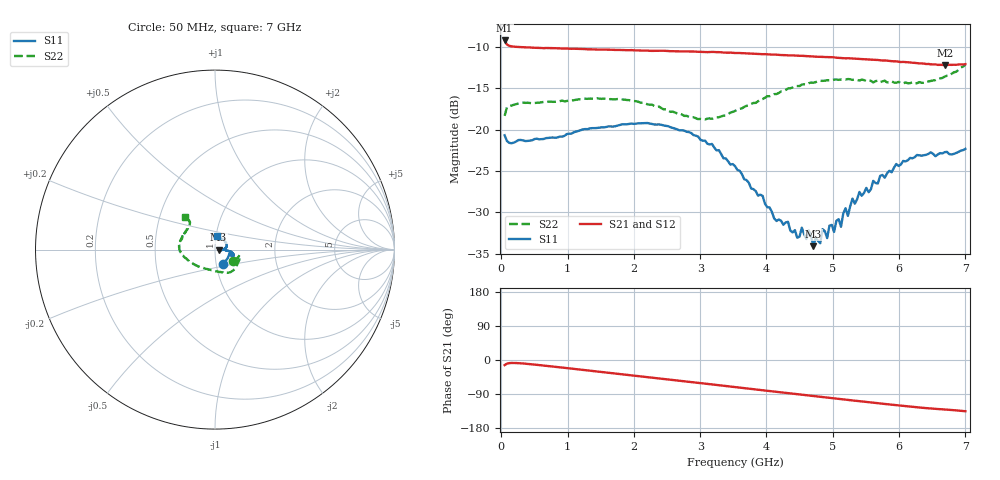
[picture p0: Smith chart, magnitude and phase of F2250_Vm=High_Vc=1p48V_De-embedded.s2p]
! Integrated Device Technology
! Corporate Headquarters
! 6024 Silver Creek Valley Road
! San Jose, CA 95138  USA
! Phone:  1-408-284-8200
! Toll Free:  1-800-223-1366
! Webpage:  http://www.idt.com/
! Timing and RF Division
! 515 Groton Road, Suite 102
! Westford, MA 01886-6024
! Device:  F2250
! Description: Voltage Variable RF Attenuator
! Frequency:  50.0 -  6000.00 MHz
! Package:  3x3 mm Thin QFN Plastic Package: 16 pin
! Ports:  2 RF, 3 DC
!  Pin  1  = GND
!  Pin  2  = NC
!  Pin  3  = RF1  = Port 1
!  Pin  4  = NC
!  Pin  5  = GND
!  Pin  6  = GND
!  Pin  7  = GND
!  Pin  8  = GND
!  Pin  9  = NC
!  Pin 10  = RF2  = Port 2
!  Pin 11  = NC
!  Pin 12  = GND
!  Pin 13  = GND
!  Pin 14  = VCNTRL
!  Pin 15  = VDD
!  Pin 16  = VMODE
! Vcntrl:  1.480 Volts
! Vmode:  +3.300 Volts
! Vdd:  +3.30  Volts
! Current:  1.331 mA
! Data:  The device was measured on a the F2250 evaluation board which has
!  individual transmission lines to the RF pins.  Data was collected
!  using a calibrated network analyzer.  The evaluation board was
!  de-embedded using a TRL calibration technique.
!  The reference plane is the edge of the package pin.
! Misc:  SN 10
!  Action Tracker AT0258
! Date Measured:  2014-11-26
! Date:  2015-10-15  MJV
! Note:
!  Integrated Device Technology supplies this data as a sample of measured
!  data at the package pin for this product.  Your particular data for this
!  product may vary.
!  Data was taken at 25 degrees C.
!  Integrated Device Technology reserves the right to change this data at anytime.
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# GHz S dB R 50
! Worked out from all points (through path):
!   201 points, 50 MHz to 7 GHz, reference 50 ohm
!   highest |S21| = -9.21 dB at 50 MHz (marker M1); lowest = -12.2 dB at 6.687 GHz (marker M2)
!   group delay of S21, straight-line fit = 53.8 ps
!   lowest |S11| = -34.1 dB at 4.707 GHz (marker M3), VSWR 1.04, Z = 52 + j0.0515 ohm
!   |S11| at or under -10 dB: start of sweep to end of sweep
!   |S22| runs from -18.8 to -12.2 dB; largest |S21 - S12| = 0.0013
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0.05  -20.67 -60.0  -9.21 -13.4  -9.21 -13.4  -18.33 -32.7
0.29325  -21.24 -13.4  -10.02 -8.8  -10.03 -8.8  -16.76 -14.7
1.2315  -19.95 -20.5  -10.24 -26.0  -10.23 -26.1  -16.24 -42.1
2.37825  -19.36 -14.7  -10.45 -48.3  -10.47 -48.3  -17.20 -69.7
2.969  -20.83 -7.4  -10.57 -60.2  -10.57 -60.2  -18.72 -97.6
3.525  -24.40 -2.8  -10.73 -71.4  -10.72 -71.5  -17.74 -132.8
4.1505  -31.04 -1.3  -10.93 -84.0  -10.94 -84.0  -15.69 -160.7
4.32425  -31.14 1.5  -11.01 -87.4  -11.01 -87.4  -15.02 -166.5
4.46325  -33.06 1.5  -11.04 -90.2  -11.06 -90.2  -14.73 -170.0
4.637  -32.15 -0.3  -11.12 -93.7  -11.12 -93.7  -14.38 -175.2
4.7065  -34.09 1.4  -11.14 -95.1  -11.16 -95.1  -14.32 -176.2
4.81075  -33.74 -7.3  -11.18 -97.1  -11.19 -97.1  -14.09 -178.3
4.8455  -32.03 -7.3  -11.20 -97.8  -11.20 -97.8  -14.10 -179.1
4.915  -33.11 -5.2  -11.21 -99.2  -11.23 -99.2  -14.02 178.8
4.94975  -31.60 -7.7  -11.22 -99.9  -11.23 -99.9  -14.01 178.1
5.1235  -31.74 -3.7  -11.32 -103.3  -11.34 -103.3  -13.92 173.9
5.15825  -30.12 -8.5  -11.35 -103.9  -11.35 -103.9  -13.90 173.5
5.22775  -30.42 -1.5  -11.36 -105.3  -11.34 -105.4  -13.87 171.6
5.29725  -28.33 -2.0  -11.37 -106.7  -11.39 -106.7  -13.98 170.2
5.85325  -24.97 5.8  -11.69 -117.2  -11.70 -117.3  -14.26 155.0
6.68725  -22.72 45.7  -12.19 -130.6  -12.18 -130.8  -13.58 132.0
7  -22.32 81.3  -12.07 -135.2  -12.09 -135.3  -12.16 132.0
